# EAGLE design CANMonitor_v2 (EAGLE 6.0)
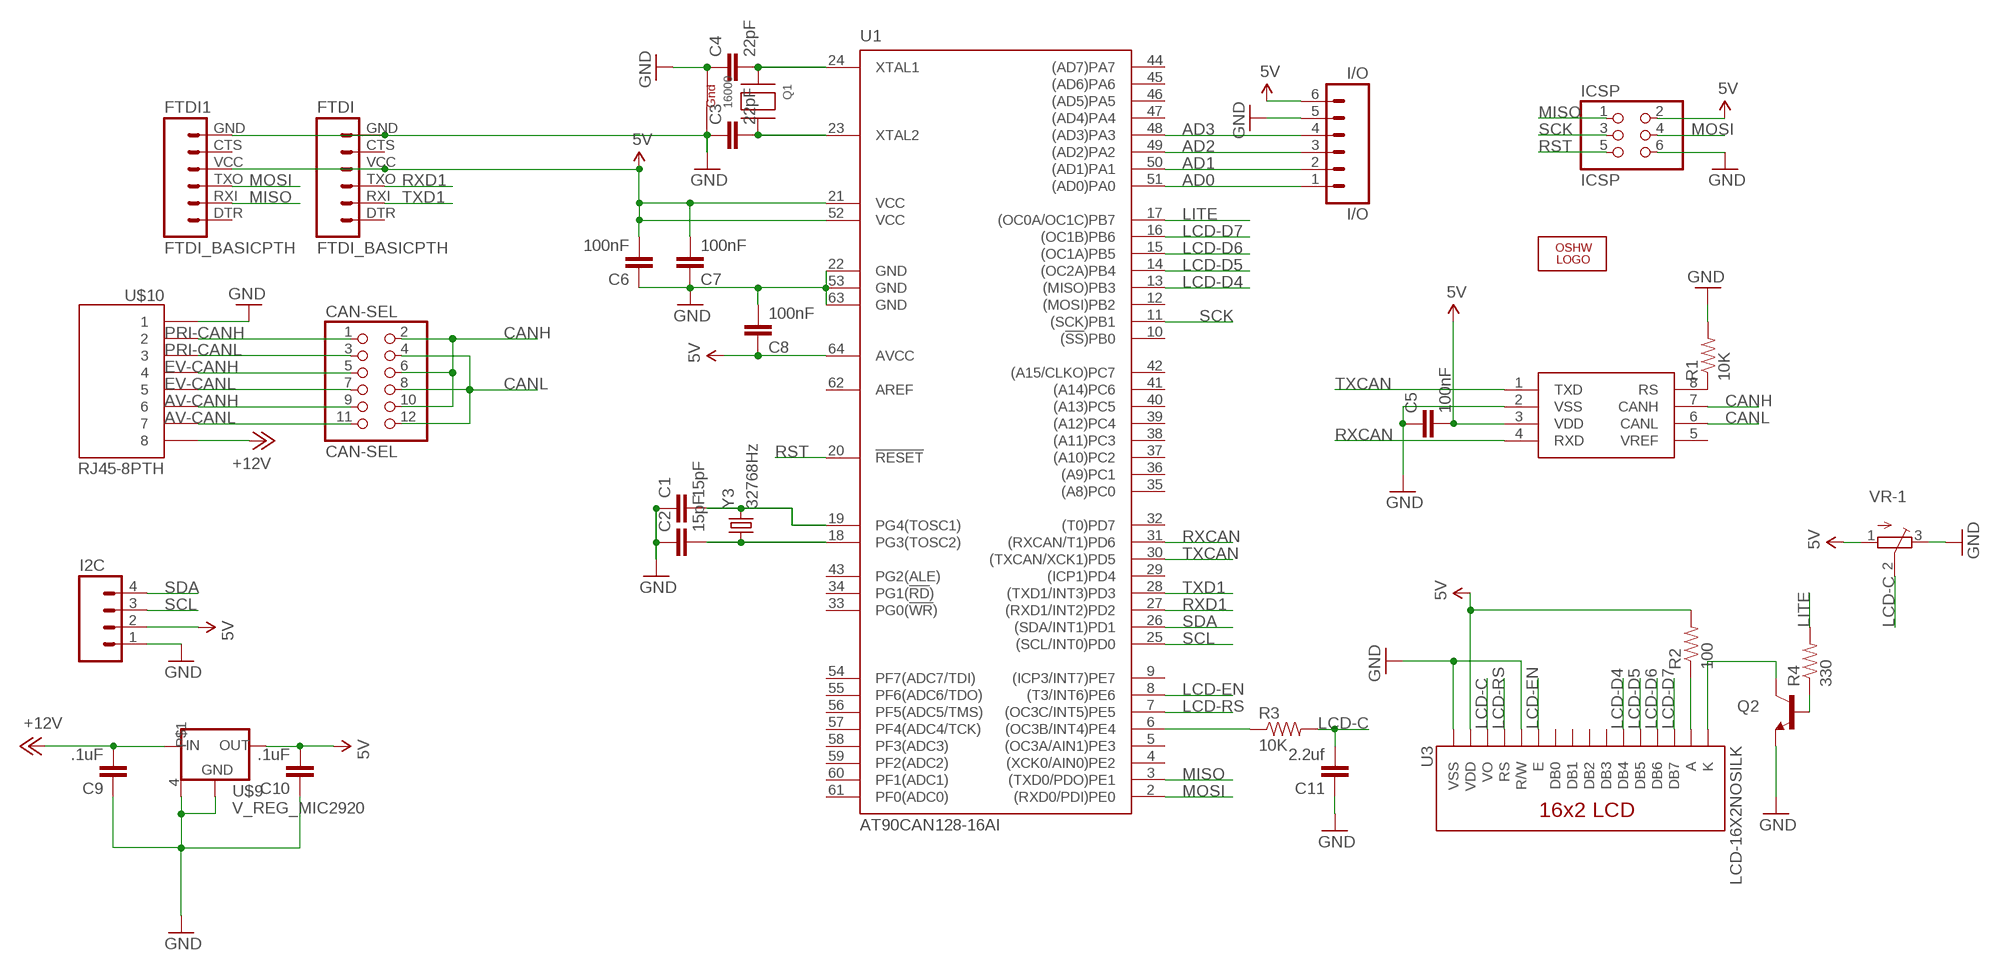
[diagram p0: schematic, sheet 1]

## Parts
C1  15pF  CAP0805  [0805]
C2  15pF  CAP0805  [0805]
C3  22pF  CAP0805  [0805]
C4  22pF  CAP0805  [0805]
C5  100nF  CAP0805  [0805]
C6  100nF  CAP0805  [0805]
C7  100nF  CAP0805  [0805]
C8  100nF  CAP0805  [0805]
C9  .1uF  CAP0805  [0805]
C10  .1uF  CAP0805  [0805]
C11  2.2uf  CAP0805  [0805]
CAN-SEL  CAN-SEL  PINHD-2X6  [2X06-BIG]
FTDI  FTDI_BASICPTH  [FTDI_BASIC]
FTDI1  FTDI_BASICPTH  [FTDI_BASIC]
I2C  M04LOCK  [1X04_LOCK]
I/O  I/O  M06LOCK  [1X06_LOCK]
ICSP  ICSP  PINHD-2X3  [2X03]
LOGO2  OSHW_LOGO_10MILX0350-NT  [OSHW_10X350_NOTEXT]
Q1  16000  XTAL-4-3225  [NX3225]
Q2  TRANSISTOR_NPNSOT23-3  [SOT23-3]
R1  10K  RESISTOR0805-RES  [0805]
R2  100  RESISTOR0805-RES  [0805]
R3  10K  RESISTOR0805-RES  [0805]
R4  330  RESISTOR0805-RES  [0805]
U1  AT90CAN128-16AI  [TQFP64-0.8MM]
U2  MCP2551  [SO08]
U3  LCD-16X2NOSILK  [LCD-16X2_NOSILK]
U$9  V_REG_MIC2920  [SOT223]
U$10  RJ45-8PTH  [RJ45-8]
VR-1  TRIMPOTTC33X  [TC33X]
Y3  32768Hz  CRYSTALTC38H  [TC38H]

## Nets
5V: C5.2 C6.2 C7.2 C8.1 C10.2 FTDI1.VCC FTDI.VCC I2C.2 I/O.6 ICSP.2 R2.2 U1.21(VCC) U1.52(VCC) U1.64(AVCC) U2.3(VDD) U3.2(VDD) U$9.3(OUT) VR-1.1(A)
+12V: C9.2 U$9.1(IN) U$10.8
AD0: I/O.1 U1.51((AD0)PA0)
AD1: I/O.2 U1.50((AD1)PA1)
AD2: I/O.3 U1.49((AD2)PA2)
AD3: I/O.4 U1.48((AD3)PA3)
AV-CANH: CAN-SEL.9 U$10.6
AV-CANL: CAN-SEL.11 U$10.7
CANH: CAN-SEL.2 CAN-SEL.6 CAN-SEL.10 U2.7(CANH)
CANL: CAN-SEL.4 CAN-SEL.8 CAN-SEL.12 U2.6(CANL)
EV-CANH: CAN-SEL.5 U$10.4
EV-CANL: CAN-SEL.7 U$10.5
GND: C1.1 C2.1 C3.1 C4.1 C5.1 C6.1 C7.1 C8.2 C9.1 C10.1 C11.1 FTDI1.GND FTDI.GND I2C.1 I/O.5 ICSP.6 Q1.1(G1) Q1.3(G2) Q2.2(E) R1.2 U1.22(GND) U1.53(GND) U1.63(GND) U2.2(VSS) U3.1(VSS) U3.5(R/W) U$9.2(GND) U$9.4 U$10.1 VR-1.3(E)
LCD-C: C11.2 R3.2 U3.3(VO) VR-1.2(S)
LCD-D4: U1.13((MISO)PB3) U3.11(DB4)
LCD-D5: U1.14((OC2A)PB4) U3.12(DB5)
LCD-D6: U1.15((OC1A)PB5) U3.13(DB6)
LCD-D7: U1.16((OC1B)PB6) U3.14(DB7)
LCD-EN: U1.8((T3/INT6)PE6) U3.6(E)
LCD-RS: U1.7((OC3C/INT5)PE5) U3.4(RS)
LITE: R4.2 U1.17((OC0A/OC1C)PB7)
MISO: FTDI1.RXI ICSP.1 U1.3((TXD0/PDO)PE1)
MOSI: FTDI1.TXO ICSP.4 U1.2((RXD0/PDI)PE0)
N$1: C2.2 U1.18(PG3(TOSC2)) Y3.1
N$2: C4.2 Q1.2(X1) U1.24(XTAL1)
N$3: C1.2 U1.19(PG4(TOSC1)) Y3.2
N$4: Q2.3(C) U3.16(K)
N$5: R1.1 U2.8(RS)
N$6: C3.2 Q1.4(X2) U1.23(XTAL2)
N$7: R3.1 U1.6((OC3B/INT4)PE4)
N$8: Q2.1(B) R4.1
N$19: R2.1 U3.15(A)
PRI-CANH: CAN-SEL.1 U$10.2
PRI-CANL: CAN-SEL.3 U$10.3
RST: ICSP.5 U1.20(!RESET)
RXCAN: U1.31((RXCAN/T1)PD6) U2.4(RXD)
RXD1: FTDI.TXO U1.27((RXD1/INT2)PD2)
SCK: ICSP.3 U1.11((SCK)PB1)
SCL: I2C.3 U1.25((SCL/INT0)PD0)
SDA: I2C.4 U1.26((SDA/INT1)PD1)
TXCAN: U1.30((TXCAN/XCK1)PD5) U2.1(TXD)
TXD1: FTDI.RXI U1.28((TXD1/INT3)PD3)
Unconnected: FTDI1.CTS FTDI1.DTR FTDI.CTS FTDI.DTR U1.4((XCK0/AIN0)PE2) U1.5((OC3A/AIN1)PE3) U1.9((ICP3/INT7)PE7) U1.10((!SS!)PB0) U1.12((MOSI)PB2) U1.29((ICP1)PD4) U1.32((T0)PD7) U1.33(PG0(!WR!)) U1.34(PG1(!RD!)) U1.35((A8)PC0) U1.36((A9)PC1) U1.37((A10)PC2) U1.38((A11)PC3) U1.39((A12)PC4) U1.40((A13)PC5) U1.41((A14)PC6) U1.42((A15/CLKO)PC7) U1.43(PG2(ALE)) U1.44((AD7)PA7) U1.45((AD6)PA6) U1.46((AD5)PA5) U1.47((AD4)PA4) U1.54(PF7(ADC7/TDI)) U1.55(PF6(ADC6/TDO)) U1.56(PF5(ADC5/TMS)) U1.57(PF4(ADC4/TCK)) U1.58(PF3(ADC3)) U1.59(PF2(ADC2)) U1.60(PF1(ADC1)) U1.61(PF0(ADC0)) U1.62(AREF) U2.5(VREF) U3.7(DB0) U3.8(DB1) U3.9(DB2) U3.10(DB3)

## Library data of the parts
C1-C11 = SparkFun:CAP: Capacitor
CAN-SEL = lincomatic:PINHD-2X6: PIN HEADER With larger annulars
FTDI FTDI1 = SparkFun:FTDI_BASIC: FTDI Basic: 3.3V and 5V
I2C = SparkFun:M04: Header 4 Standard 4-pin 0.1" header. Use with straight break away headers (SKU : PRT-00116), right angle break away headers (PRT-00553), swiss pins (PRT-00743), machine pins (PRT-00117), and female headers (PRT-00115). Molex polarized connector foot print use with SKU : PRT-08231 with associated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
I/O = SparkFun:M06: Header 6 Standard 6-pin 0.1" header. Use with straight break away headers (SKU : PRT-00116), right angle break away headers (PRT-00553), swiss pins (PRT-00743), machine pins (PRT-00117), and female headers (PRT-00115). Molex polarized connector foot print use with SKU : PRT-08094 with associated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
ICSP = SparkFun:PINHD-2X3: PIN HEADER
LOGO2 = ohw-logo:OSHW_LOGO_10MIL
Q1 = adafruit:XTAL-4: Classic 4-pin 3.2 x 2.5mm crystal
Q2 = SparkFun:TRANSISTOR_NPN: Transistor NPN BJT configuration in SOT23 package. MMBT2222 is the common NPN we use. Double check BCE configuration again layout.
R1-R4 = SparkFun:RESISTOR: Resistor
U1 = _hhn_at90can32_64_128_v2:AT90CAN*: ATMEL AVR AT90CAN32-..A. / 64-..A. / 128-..A., TQFP64 with 0.8mm pad spacing (Atmel Package Code 'A2 64': 64-Lead, Thin 1.0 mm / 0.03937 in. Plastic Gull Wing Quad Flat Package) Ordering Code = Product Marking / Speed (MHz) / Power Supply (V) / Operation Range AT90CANx-16AI / 16 / 2.7 .. 5.5 /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
U2 = SparkFun:MCP2551
U3 = SparkFun:LCD-16X2
U$9 = SparkFun:V_REG_MIC2920: MIC2920A (http://www.micrel.com/_PDF/mic2920.pdf) - 400mA output LDO Regulator
U$10 = SparkFun:RJ45-8: RJ45 Jack Simple RJ45, 8-pin connection - connector for common Cat5, Cat5e, and Cat6 Ethernet cables. Footprint not yet proven in production. Connector sku is PRT-00643; Breakout PCB sku is BOB-00716.
VR-1 = adafruit:TRIMPOT: SMT trimmer potentiometer part number TC33X http://www.ladyada.net/library/eagle
Y3 = SparkFun:CRYSTAL: Crystals

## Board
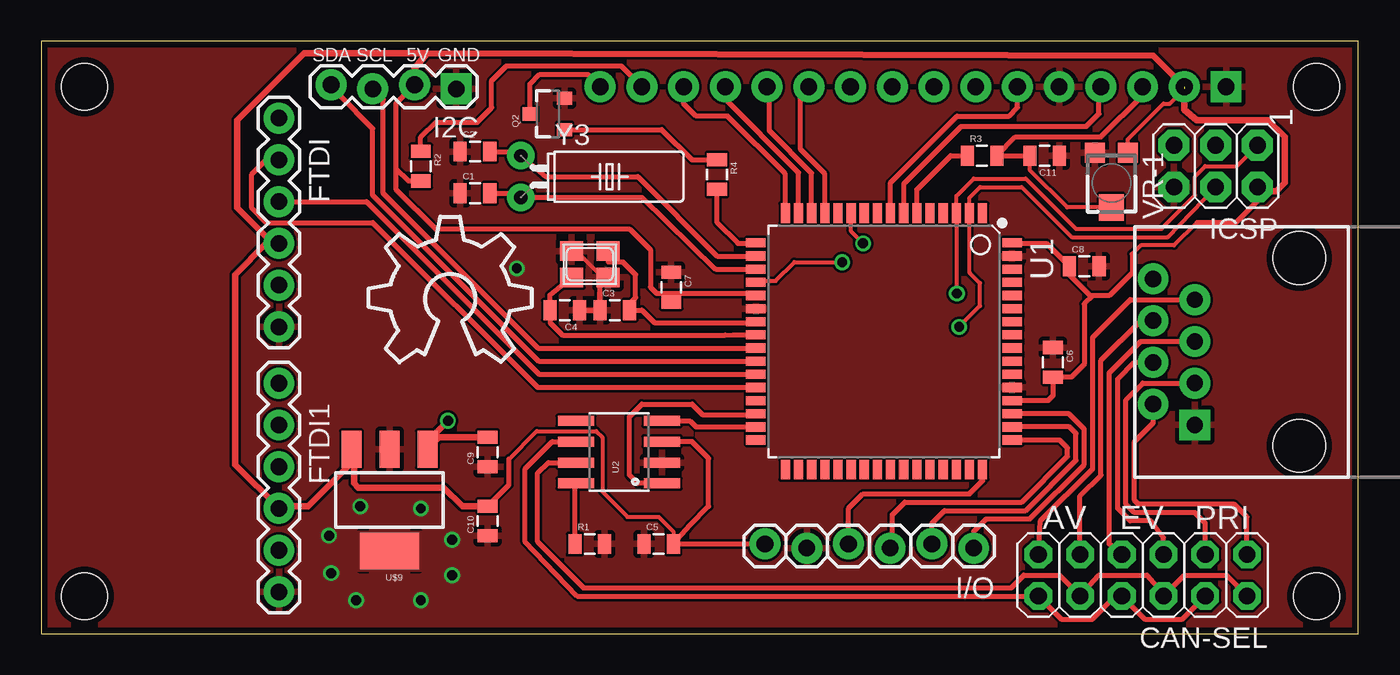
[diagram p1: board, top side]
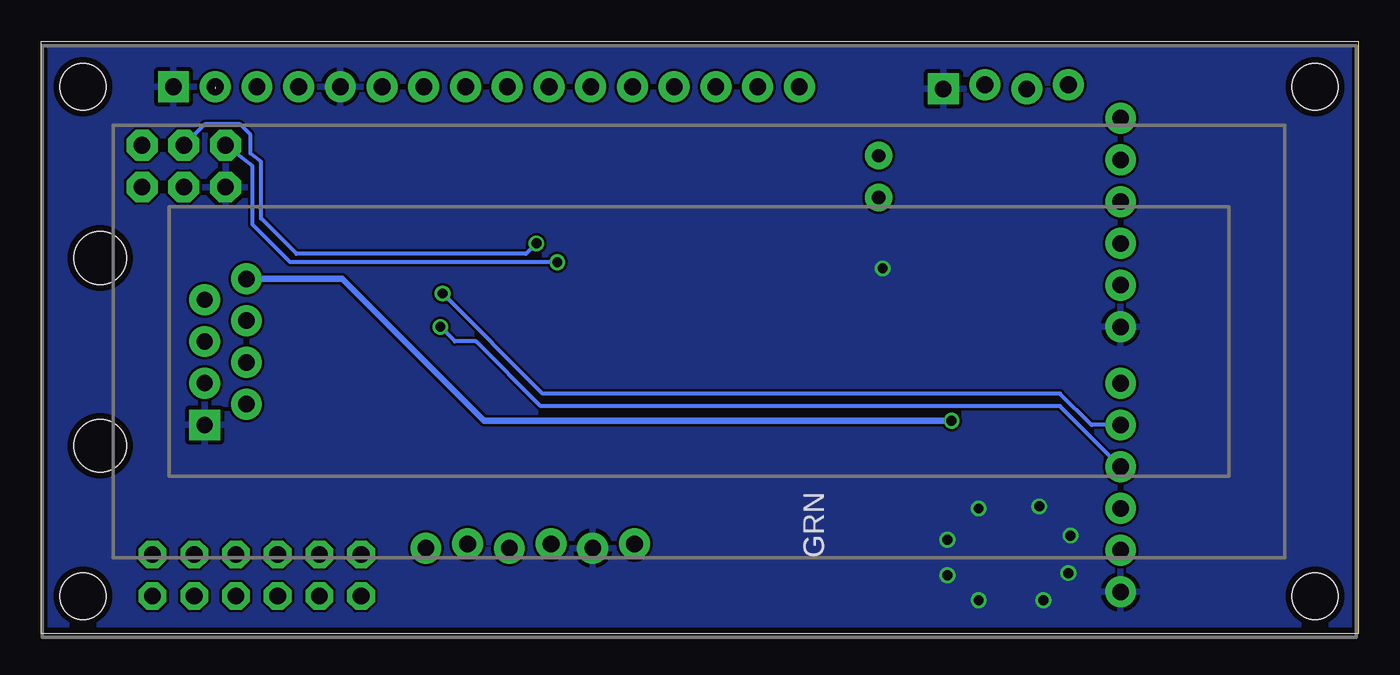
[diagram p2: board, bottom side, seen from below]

Size 80.19 x 36.06 mm. Coordinates in mm from the lower left corner, seen from the top.
Outline: 0,0 80.19,0 80.19,36.06 0,36.06 0,0
Copper layers (1*16): Top 0.0356mm / dielectric 1.5011mm / Bottom 0.0356mm
Design rules: minimum track width 6mil, minimum drill 13mil, track to track 6mil, track to pad 6mil, pad to pad 6mil, via to via 6mil, smd to smd 6mil, copper to edge 15mil, drill to drill 6mil, minimum pad ring 7mil, minimum via ring 7mil, stop-mask expansion 4mil, vias tented up to drill 0mil, thermal gap 10mil

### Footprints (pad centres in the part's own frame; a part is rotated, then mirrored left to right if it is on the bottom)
0805 = smd 0.8 x 1.2: 1 -0.9,0; 2 0.9,0
2X06-BIG = drill 1.016 pad 1.676 octagon: 1 -6.35,-1.27; 2 -6.35,1.27; 3 -3.81,-1.27; 4 -3.81,1.27; 5 -1.27,-1.27; 6 -1.27,1.27; 7 1.27,-1.27; 8 1.27,1.27; 9 3.81,-1.27; 10 3.81,1.27; 11 6.35,-1.27; 12 6.35,1.27
FTDI_BASIC = drill 1.016 pad 1.88: CTS 10.16,0; DTR 0,0; GND 12.7,0; RXI 2.54,0; TXO 5.08,0; VCC 7.62,0
1X04_LOCK = drill 1.016 pad 1.88 square: 1 0,0.127 | drill 1.016 pad 1.88: 2 2.54,-0.127; 3 5.08,0.127; 4 7.62,-0.127
1X06_LOCK = drill 1.016 pad 1.88: 1 0,0; 2 2.54,-0.254; 3 5.08,0; 4 7.62,-0.254; 5 10.16,0; 6 12.7,-0.254
2X03 = drill 1.016 pad 1.88 octagon: 1 -2.54,-1.27; 2 -2.54,1.27; 3 0,-1.27; 4 0,1.27; 5 2.54,-1.27; 6 2.54,1.27
NX3225 = smd 1.4 x 1.2: 1 -1.1,0.8; 2 1.1,0.8; 3 1.1,-0.8; 4 -1.1,-0.8
SOT23-3 = smd 0.8 x 0.9: 1 -0.95,-1; 2 0.95,-1; 3 0,1.1
TQFP64-0.8MM = smd 1.194 x 0.559: 1 -7.8,6; 2 -7.8,5.2; 3 -7.8,4.4; 4 -7.8,3.6; 5 -7.8,2.8; 6 -7.8,2; 7 -7.8,1.2; 8 -7.8,0.4; 9 -7.8,-0.4; 10 -7.8,-1.2; 11 -7.8,-2; 12 -7.8,-2.8; 13 -7.8,-3.6; 14 -7.8,-4.4; 15 -7.8,-5.2; 16 -7.8,-6; 33 7.8,-6; 34 7.8,-5.2; 35 7.8,-4.4; 36 7.8,-3.6; 37 7.8,-2.8; 38 7.8,-2; 39 7.8,-1.2; 40 7.8,-0.4; 41 7.8,0.4; 42 7.8,1.2; 43 7.8,2; 44 7.8,2.8; 45 7.8,3.6; 46 7.8,4.4; 47 7.8,5.2; 48 7.8,6 | smd 0.559 x 1.194: 17 -6,-7.8; 18 -5.2,-7.8; 19 -4.4,-7.8; 20 -3.6,-7.8; 21 -2.8,-7.8; 22 -2,-7.8; 23 -1.2,-7.8; 24 -0.4,-7.8; 25 0.4,-7.8; 26 1.2,-7.8; 27 2,-7.8; 28 2.8,-7.8; 29 3.6,-7.8; 30 4.4,-7.8; 31 5.2,-7.8; 32 6,-7.8; 49 6,7.8; 50 5.2,7.8; 51 4.4,7.8; 52 3.6,7.8; 53 2.8,7.8; 54 2,7.8; 55 1.2,7.8; 56 0.4,7.8; 57 -0.4,7.8; 58 -1.2,7.8; 59 -2,7.8; 60 -2.8,7.8; 61 -3.6,7.8; 62 -4.4,7.8; 63 -5.2,7.8; 64 -6,7.8
SO08 = smd 0.61 x 2.21: 1 -1.905,-2.616; 2 -0.635,-2.616; 3 0.635,-2.616; 4 1.905,-2.616; 5 1.905,2.616; 6 0.635,2.616; 7 -0.635,2.616; 8 -1.905,2.616
LCD-16X2_NOSILK = drill 1.016 pad 1.88 square: 1 -32,15.5 | drill 1.016 pad 1.88: 2 -29.46,15.5; 3 -26.92,15.5; 4 -24.38,15.5; 5 -21.84,15.5; 6 -19.3,15.5; 7 -16.76,15.5; 8 -14.22,15.5; 9 -11.68,15.5; 10 -9.14,15.5; 11 -6.6,15.5; 12 -4.06,15.5; 13 -1.52,15.5; 14 1.02,15.5; 15 3.56,15.5; 16 6.1,15.5 | hole 2.8: -37.5,15.5; -37.5,-15.5; 37.5,15.5; 37.5,-15.5
SOT223 = smd 1.219 x 2.235: 1 -2.311,-3.099; 2 0,-3.099; 3 2.311,-3.099 | smd 3.6 x 2.2: 4 0,3.099
RJ45-8 = drill 1 pad 1.88 square: 1 -4.445,6.35 | drill 1 pad 1.88: 2 -3.175,8.89; 3 -1.905,6.35; 4 -0.635,8.89; 5 0.635,6.35; 6 1.905,8.89; 7 3.175,6.35; 8 4.445,8.89 | hole 3.2: -5.715,0; 5.715,0
TC33X = smd 1.2 x 1.2: 1 -1,-1.825; 3 1,-1.825 | smd 1.5 x 1.6: 2 0,1.5
TC38H = drill 0.813 pad 1.676: 1 -1.27,0; 2 1.27,0

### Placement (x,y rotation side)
C1  26.42,26.8 0 top
C2  26.42,29.34 0 top
C3  34.92,19.68 0 top
C4  31.88,19.68 180 top
C5  37.59,5.46 0 top
C6  61.59,16.51 270 top
C7  38.35,21.08 270 top
C8  63.5,22.35 0 top
C9  27.18,11.05 90 top
C10  27.18,6.86 90 top
C11  61.09,29.08 180 top
CAN-SEL  67.06,3.56 180 top
FTDI  14.48,31.37 270 top
FTDI1  14.48,15.24 270 top
I2C  25.27,33.27 180 top
I/O  56.77,5.21 180 top
ICSP  71.5,28.45 180 top
LOGO2  19.94,16.51 0 top
Q1  33.4,22.48 180 top
Q2  30.86,31.62 90 top
R1  33.4,5.46 0 top
R2  23.11,28.45 270 top
R3  57.28,29.08 0 top
R4  41.15,27.94 270 top
U1  51.31,17.78 270 top
U2  35.18,11.05 90 top
U3  40.13,17.78 0 bottom
U$9  21.21,8.13 180 top
U$10  76.58,17.14 90 top
VR-1  65.15,27.43 180 top
Y3  29.21,27.81 270 top

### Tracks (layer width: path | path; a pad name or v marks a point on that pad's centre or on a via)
5V  (1 unrouted)
  Top 0.254: 28.47,10.62 30.18,12.32 33.78,12.32 34.16,11.94 34.16,8.64 35.69,7.11 37.59,7.11 38.49,6.21 C5.2 | 70.36,25.02 68.96,23.62 66.93,23.62 66.42,23.11 | VR-1.1 66.15,30.08 68.33,32.26 68.71,32.26 69.6,33.15
  Top 0.305: 59.08,23.75 U1.64 59.15,23.74 61.21,23.74 C8.1 62.6,21.86 63.88,20.57 64.01,20.57 | U1.21 43.39,20.7 38.09,20.7 | 38.09,20.7 C7.2 | 38.09,20.7 37.47,20.7 37.08,21.08 37.08,23.37 35.81,24.64 24,24.64 21.59,27.05 21.59,28.32 | 64.01,20.57 65.02,20.57 66.42,21.97 66.42,23.11 | 70.36,25.02 72.74,25.02 74.22,26.5 | U1.52 61.3,14.18 61.59,14.48 C6.2 62.73,15.61 63.5,16.38 63.5,20.07 64.01,20.57 | U2.3 39.62,11.68 40.64,10.67 40.64,7.75 39.5,6.6 C5.2 I/O.6 | C10.2 28.47,9.05 28.47,10.62 | R2.2 22.36,27.55 21.59,28.32 | 21.59,28.32 21.59,32.26 I2C.2
  Top 0.406: 23.5,35.31 22.73,34.42 I2C.2 22.73,33.53 | 23.5,35.31 67.69,35.18 U3.2 69.59,31.88 70.36,31.24 74.68,31.24 75.69,30.23 75.69,27.43 75.18,26.92 74.3,26.92 ICSP.2 74.22,26.5 | 23.5,35.31 16,35.31 11.94,31.24 11.94,25.91 14.1,23.75 FTDI.VCC 13.72,23.75 11.81,21.84 11.81,10.29 FTDI1.VCC 14.61,7.75 16.26,7.75 18.9,10.39 U$9.3 19.05,11.07 19.05,9.14 19.3,8.89 24.51,8.89 25.64,7.76 C10.2
+12V  (via drill 0.6)
  Top 0.406: v24.77,12.95 23.52,11.71 U$9.1 24.24,11.95 C9.2
  Bottom 0.406: v24.77,12.95 53.21,12.95 61.85,21.59 U$10.8
AD0
  Top 0.305: U1.51 62.57,13.38 63.5,12.45 63.5,10.29 60.2,6.99 57.53,6.99 56.77,6.22 I/O.1
AD1
  Top 0.305: U1.50 62.6,12.58 62.99,12.19 62.99,10.54 59.94,7.49 54.99,7.49 54.23,6.73 I/O.2
AD2
  Top 0.305: U1.49 62.01,11.78 62.48,11.3 62.48,10.79 59.69,8 52.58,8 51.82,7.24 51.82,5.33 I/O.3
AD3
  Top 0.305: U1.48 57.31,9.3 56.52,8.51 50.04,8.51 49.15,7.62 I/O.4
AV-CANH
  Top 0.305: U$10.6 66.93,19.05 64.52,16.64 64.52,9.65 63.25,8.38 CAN-SEL.9
AV-CANL
  Top 0.305: U$10.7 66.29,20.32 64.01,18.03 64.01,10.03 60.83,6.86 CAN-SEL.11
CANH
  Top 0.305: CAN-SEL.2 72.14,3.56 69.6,3.56 CAN-SEL.6 68.33,2.41 67.31,3.56 64.39,3.56 CAN-SEL.10 61.98,3.56 59.82,3.56 59.05,2.79 33.02,2.79 30.23,5.59 30.23,9.78 30.86,10.41 U2.7
CANL
  Top 0.305: CAN-SEL.4 69.47,0.89 67.18,0.89 CAN-SEL.8 65.41,2.29 64.01,0.89 62.1,0.89 CAN-SEL.12 32.64,2.29 29.46,5.59 29.46,10.03 31.11,11.68 U2.6
EV-CANH
  Top 0.305: U$10.4 66.55,16.51 65.53,15.49 65.53,7.62 66.29,6.86 67.56,6.86 68.33,5.84 CAN-SEL.5
EV-CANL
  Top 0.305: U$10.5 66.93,17.78 65.02,15.88 65.02,5.46 CAN-SEL.7
GND  (via drill 0.6)
  Top 0.254: 32.51,23.37 34.04,21.84 34.34,21.84 Q1.1
  Top 0.305: 34.33,21.68 Q1.1 34.02,21.2 C3.1 C4.1 | 32.51,23.37 32.21,23.24 Q1.3
  other vias: 23.11,7.62 17.65,3.68 23.11,2.03 19.18,2.03 25.02,3.56 25.02,5.71 19.43,7.75 17.53,5.97 28.96,22.23
  pour Top: -8.64,-13.97 94.23,-13.97 94.23,53.34 -8.64,53.34
  pour Bottom: -6.35,-5.84 86.11,-5.84 86.11,43.94 -6.35,43.94 -6.35,-5.08
  pour Top: 19.18,6.6 23.62,6.6 23.62,3.56 18.92,3.56 18.92,6.6
LCD-C
  Top 0.254: VR-1.2 62.46,25.93 60.2,28.19 C11.2
  Top 0.305: U3.3 67.05,32.76 64.52,30.23 59.32,30.23 R3.2 C11.2
LCD-D4
  Top 0.305: U1.13 47.71,27.98 46.23,29.46 46.23,32.78 U3.11
LCD-D5
  Top 0.305: U1.14 46.91,28.02 44.32,30.61 44.32,33.15 U3.12
LCD-D6
  Top 0.305: U1.15 46.11,28.06 41.53,32.64 41.53,33.16 U3.13
LCD-D7
  Top 0.305: U1.16 45.31,27.97 41.78,31.5 39.88,31.5 39.12,32.26 U3.14
LCD-EN
  Top 0.305: U1.8 51.71,27.45 55.75,31.5 58.93,31.5 59.44,32 U3.6
LCD-RS
  Top 0.305: U1.7 52.51,27.36 56.01,30.86 63.63,30.86 64.39,31.62 64.39,33.16 U3.4
LITE
  Top 0.305: R4.2 41.15,25.02 42.42,23.75 43.48,23.75 U1.17
MISO  (via drill 0.6)
  Top 0.254: ICSP.1 72.77,28.45 70.87,28.45 70.23,27.81 70.23,26.67 68.2,24.64 62.99,24.64 59.94,27.69 56.77,27.69 55.71,26.62 U1.3 55.75,25.54 v55.75,20.7
  Bottom 0.254: v55.75,20.7 49.66,14.61 18.16,14.61 16.26,12.7 FTDI1.RXI
MOSI  (via drill 0.6)
  Top 0.254: ICSP.4 68.58,24.13 62.74,24.13 59.69,27.18 57.15,27.18 56.51,26.54 U1.2 56.52,21.97 57.15,21.34 57.15,19.94 v55.88,18.67
  Bottom 0.254: v55.88,18.67 54.99,17.78 53.72,17.78 49.78,13.84 18.16,13.84 FTDI1.TXO
N$1
  Top 0.305: U1.18 41.16,22.98 36.32,27.81 30.73,27.81 Y3.1 29.46,29.08 29.46,29.34 C2.2
N$2
  Top 0.305: 43.49,18.16 U1.24 42.15,18.18 41.66,18.16 31.74,18.16 30.99,18.91 C4.2 30.98,20.61 Q1.2
N$3
  Top 0.305: U1.19 41.07,22.18 36.58,26.54 Y3.2 29.34,26.54 29.34,26.8 C1.2
N$4
  Top 0.305: Q2.3 29.76,33.44 30.35,34.04 33.28,34.04 U3.16
N$5
  Top 0.305: R1.1 32.5,9.08 U2.8
N$6
  Top 0.305: Q1.4 34.54,22.61 35.43,22.61 36.2,21.84 36.2,20.45 35.83,20.08 C3.2 36.58,19.68 37.34,18.92 43.45,18.92 U1.23
N$7
  Top 0.305: U1.6 53.31,27.02 55.37,29.08 R3.1
N$8
  Top 0.305: Q2.1 37.78,30.67 39.62,28.83 41.14,28.83 R4.1
N$19
  Top 0.305: U3.15 35.31,34.54 28.32,34.54 27.43,33.66 27.43,32 26.54,31.11 24,31.11 23.11,30.23 R2.1
PRI-CANH
  Top 0.305: U$10.2 67.69,12.83 66.55,11.68 66.55,8.13 66.8,7.87 72.64,7.87 73.41,7.11 CAN-SEL.1
PRI-CANL
  Top 0.305: U$10.3 67.06,15.24 66.04,14.22 66.04,7.87 66.55,7.37 70.23,7.37 70.87,6.73 CAN-SEL.3
RST  (via drill 0.6)
  Top 0.254: v48.77,22.61 45.85,22.61 44.7,21.46 43.59,21.46 U1.20
  Bottom 0.254: v48.77,22.61 65.02,22.61 67.31,24.89 67.31,28.45 ICSP.5
RXCAN
  Top 0.305: U1.31 39.87,12.58 39.5,12.95 U2.4
RXD1
  Top 0.305: U1.27 30.32,15.78 19.81,26.29 FTDI.TXO
SCK  (via drill 0.6)
  Top 0.254: U1.11 49.31,24.48 v50.04,23.75
  Bottom 0.254: v50.04,23.75 50.67,23.11 64.64,23.11 66.8,25.27 66.8,28.7 67.44,29.21 67.44,30.35 68.07,30.99 70.23,30.99 ICSP.3
SCL
  Top 0.305: U1.25 30.25,17.38 20.83,26.8 20.83,32.51 I2C.3
SDA
  Top 0.305: U1.26 30.28,16.58 20.19,26.67 20.19,30.73 18.16,32.77 18.16,32.89 I2C.4
TXCAN
  Top 0.305: 43.46,13.34 40.26,13.34 39.62,13.97 36.58,13.97 35.81,13.21 35.81,9.65 36.32,9.14 U2.1 38.48,9.14
  Top 0.406: 43.46,13.34 U1.30
TXD1
  Top 0.305: U1.28 30.23,14.98 20.19,25.02 13.72,25.02 12.83,25.91 12.83,27.94 13.72,28.83 FTDI.RXI

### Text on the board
tNames: SDA | SCL | 5V | GND | 1 | AV | EV | PRI
bNames: GRN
